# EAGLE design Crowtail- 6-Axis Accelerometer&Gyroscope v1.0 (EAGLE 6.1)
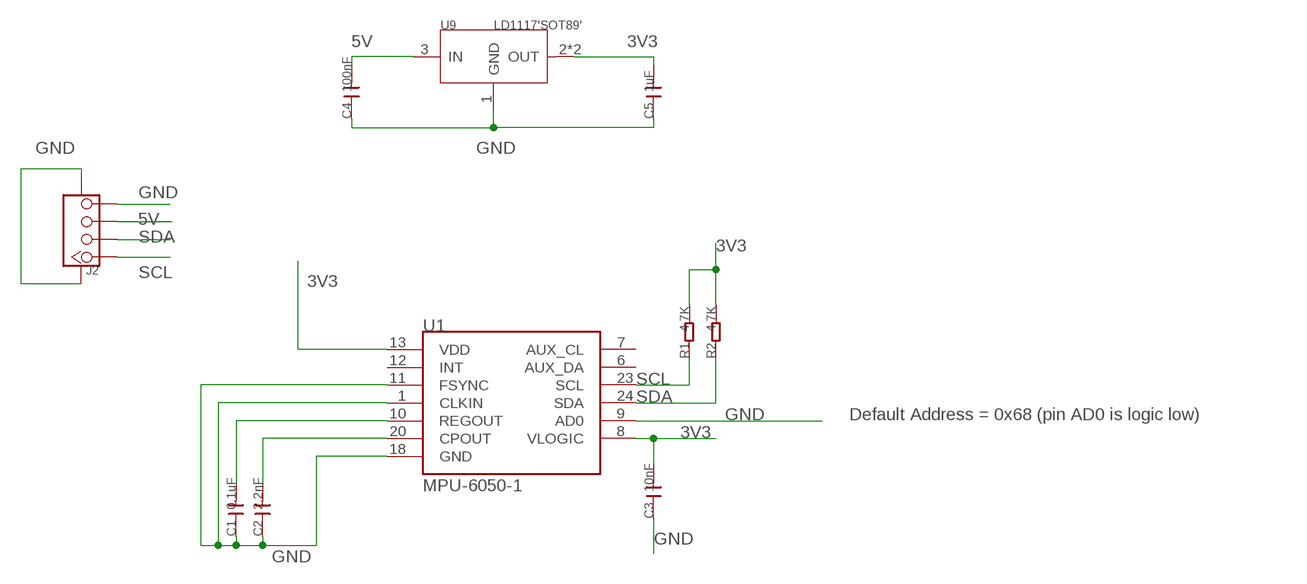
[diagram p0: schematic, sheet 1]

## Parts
C1  0.1uF  C-0603  [C0603]
C2  2.2nF  C-0603  [C0603]
C3  10nF  C-0603  [C0603]
C4  100nF  C-0603  [C0603]
C5  1uF  C-0603  [C0603]
J2  TWIG-4P-2.0-SMD-FEMALE-REINFORCE'DD'  [4P-SMD-2.0]
R1  4.7K  R-0603  [R0603]
R2  4.7K  R-0603  [R0603]
U1  MPU-6050-1  [QFN-24-4MM2]
U9  LD1117'SOT89'  [SOT89]

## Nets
3V3: C3.2 C5.2 R1.2 R2.2 U1.8(VLOGIC) U1.13(VDD) U9.2(OUT) U9.4(OUT)
5V [usbvcc]: C4.2 J2.3 U9.3(IN)
GND: C1.1 C2.1 C3.1 C4.1 C5.1 J2.4 J2.SS1 J2.SS2 U1.1(CLKIN) U1.9(AD0) U1.11(FSYNC) U1.18(GND) U9.1(GND)
N$2: C1.2 U1.10(REGOUT)
N$3: C2.2 U1.20(CPOUT)
SCL: J2.1 R1.1 U1.23(SCL)
SDA: J2.2 R2.1 U1.24(SDA)
Unconnected: U1.6(AUX_DA) U1.7(AUX_CL) U1.12(INT)

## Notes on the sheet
- Default Address = 0x68 (pin AD0 is logic low)

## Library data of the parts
C1-C5 = Discrete:C*: Ceramic Capacitors
J2 = Connector:TWIG-4P-2.0-SMD-FEMALE-REINFORCE
R1 R2 = Discrete:R*
U1 = Testing:MPU-6050
U9 = IC:LD1117: Low Drop Fixed And Adjustable Positive Voltage Regulators http://www.datasheetcatalog.org/datasheet/SGSThomsonMicroelectronics/mXuqtqv.pdf

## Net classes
0 default: width 0.203 mm
3 usbvcc: width 0.508 mm, drill 0.61 mm, clearance 0.254 mm

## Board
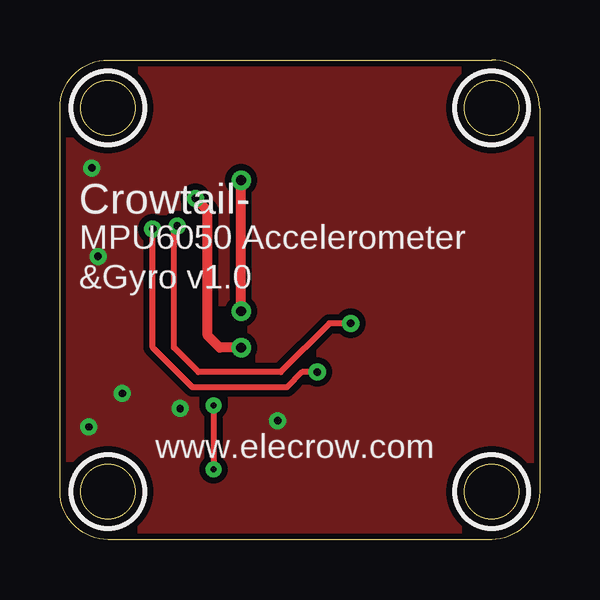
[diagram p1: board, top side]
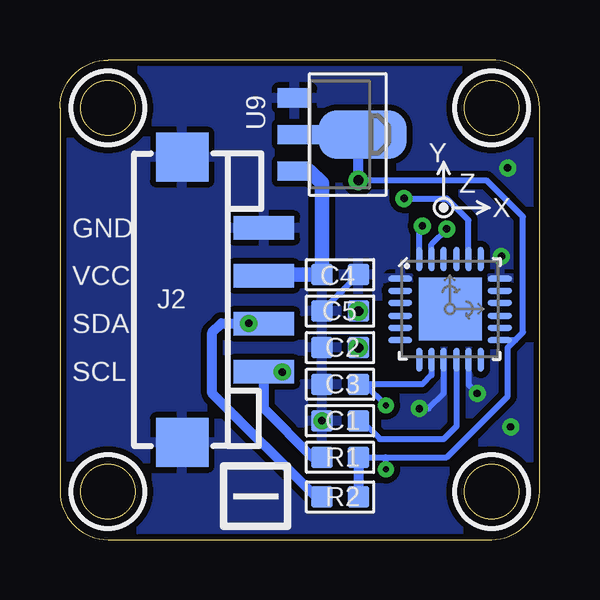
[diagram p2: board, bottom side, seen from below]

Size 20 x 20 mm. Coordinates in mm from the lower left corner, seen from the top.
Outline: 20,18 20,2 arc-90 18,0 2,0 arc-90 0,2 0,18 arc-90 2,20 18,20 arc-90 20,18
Outline: circle at 18,18 radius 1.14
Outline: circle at 18,2 radius 1.14
Outline: circle at 2,18 radius 1.14
Outline: circle at 2,2 radius 1.14
Copper layers (1*16): Top 0.035mm / dielectric 1.5mm / Bottom 0.035mm
Design rules: minimum track width 10mil, minimum drill 10mil, track to track 8mil, track to pad 8mil, pad to pad 8mil, via to via 8mil, smd to smd 0mil, copper to edge 10mil, drill to drill 8mil, minimum pad ring 10mil, minimum via ring 8mil, stop-mask expansion 4mil, vias tented up to drill 100mil, thermal gap 10mil
tRestrict: area 16.5,16.5 to 19.5,19.5; area 16.5,0.5 to 19.5,3.5; area 0.5,16.5 to 3.5,19.5; area 0.5,0.5 to 3.5,3.5
bRestrict: area 16.5,16.5 to 19.5,19.5; area 16.5,0.5 to 19.5,3.5; area 0.5,16.5 to 3.5,19.5; area 0.5,0.5 to 3.5,3.5

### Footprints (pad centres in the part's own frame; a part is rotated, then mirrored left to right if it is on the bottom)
C0603 = smd 0.889 x 0.889: 1 -0.762,0; 2 0.762,0
4P-SMD-2.0 = smd 0.965 x 2.54: 1 -3,0; 2 -1,0; 3 1,0; 4 3,0 | smd 2.032 x 2.184: SS1 -5.946,3.4; SS2 5.946,3.4
R0603 = smd 0.889 x 0.889: 1 -0.762,0; 2 0.762,0
QFN-24-4MM2 = smd 1.016 x 0.254: 1 -2.066,1.257; 2 -2.066,0.75; 3 -2.066,0.247; 4 -2.066,-0.287; 5 -2.066,-0.792; 6 -2.066,-1.297; 13 2.086,-1.297; 14 2.086,-0.792; 15 2.086,-0.287; 16 2.086,0.247; 17 2.086,0.75; 18 2.086,1.257 | smd 0.254 x 1.016: 7 -1.267,-2.122; 8 -0.762,-2.122; 9 -0.258,-2.122; 10 0.278,-2.122; 11 0.78,-2.122; 12 1.287,-2.122; 19 1.287,2.082; 20 0.78,2.082; 21 0.278,2.082; 22 -0.258,2.082; 23 -0.762,2.082; 24 -1.267,2.082 | smd 2.616 x 2.616: P$1 0.02,-0.01
SOT89 = smd 0.8 x 1.4: 1 -1.524,-1.905; 3 1.524,-1.905 | smd 0.8 x 1.9: 2 0,-1.651 | smd 2.032 x 3.65: 4 0,0.94

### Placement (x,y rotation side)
C1  8.32,4.95 0 bottom
C2  8.32,8 0 bottom
C3  8.32,6.48 0 bottom
C4  8.32,11.05 180 bottom
C5  8.32,9.53 0 bottom
J2  11.5,10 90 bottom
R1  8.32,3.43 0 bottom
R2  8.32,1.78 0 bottom
U1  3.74,9.62 0 bottom
U9  8.32,16.89 270 bottom

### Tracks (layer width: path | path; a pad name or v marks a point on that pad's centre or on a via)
3V3  (via drill 0.25, 0.41)
  Top 0.254: v6.41,5.59 v6.41,2.92
  Top 0.406: C5.2 v7.55,14.99
  Bottom 0.254: R1.2 6.41,3.43 | 6.41,3.43 3.87,3.43 1.33,5.97 1.33,8 1.01,8.32 | v7.55,14.99 2.22,14.99 0.7,13.46 0.7,8.64 1.01,8.32 | U1.13 1.01,8.32 | v6.41,5.59 7.3,6.48 C3.2 4.89,6.48 4.51,6.86 U1.8 | v6.41,2.92 6.41,3.43
  Bottom 0.406: R1.2 R2.2 | v7.55,14.99 7.55,16.71
  Bottom 0.61: 7.55,16.71 U9.4 U9.2
  other vias: 7.55,9.53
5V
  Bottom 0.61: J2.3 11.45,11.05 C4.2 9.08,14.86 9.59,15.37 U9.3
GND  (via drill 0.3)
  Bottom 0.254: C5.1 C4.1 | U1.9 4,6.1 4.63,5.46 v5.01,5.46 | U1.11 2.96,6.46 v2.6,6.1
  other vias: 1.2,4.7 1.33,15.49 1.58,11.81 9.08,4.95
  pour Top (isolate 0.254): 20.51,-0.76 -0.45,-0.89 -0.32,20.32 20.64,20.45
  pour Bottom (isolate 0.254): 20.51,-0.89 -0.45,-0.89 -0.32,20.45 20.64,20.45
N$2
  Bottom 0.254: U1.10 3.47,4.72 4,4.19 6.67,4.19 7.43,4.95 C1.2
N$3  (via drill 0.3, 0.41)
  Top 0.406: C2.2 6.67,8 6.16,8.51 6.16,13.72 v5.65,14.22
  Bottom 0.254: v5.65,14.22 3.87,14.22 2.96,13.32 U1.20
  other vias: 7.55,8
SCL  (via drill 0.3)
  Top 0.254: v10.73,6.99 10.09,6.99 9.46,6.35 5.52,6.35 3.87,8 v3.87,12.95
  Bottom 0.254: J2.1 v10.73,6.99 | v3.87,12.95 4.51,12.32 U1.23
  Bottom 0.406: R1.1 9.46,3.43 11.49,5.46 J2.1
SDA  (via drill 0.3)
  Top 0.254: v12.13,9.02 11.24,9.02 9.21,6.99 5.78,6.99 4.76,8 4.76,12.95 v4.89,13.08
  Bottom 0.254: J2.2 12.11,9 v12.13,9.02 | U1.24 5.01,12.96 v4.89,13.08
  Bottom 0.406: R2.1 9.33,1.78 13.65,6.1 13.65,8.64 13.27,9.02 v12.13,9.02 11.52,9.02 J2.2

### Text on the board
tPlace: Crowtail- | MPU6050 Accelerometer | &Gyro v1.0 | www.elecrow.com
bPlace: GND | VCC | SDA | SCL | I
bNames: Y | Z | X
